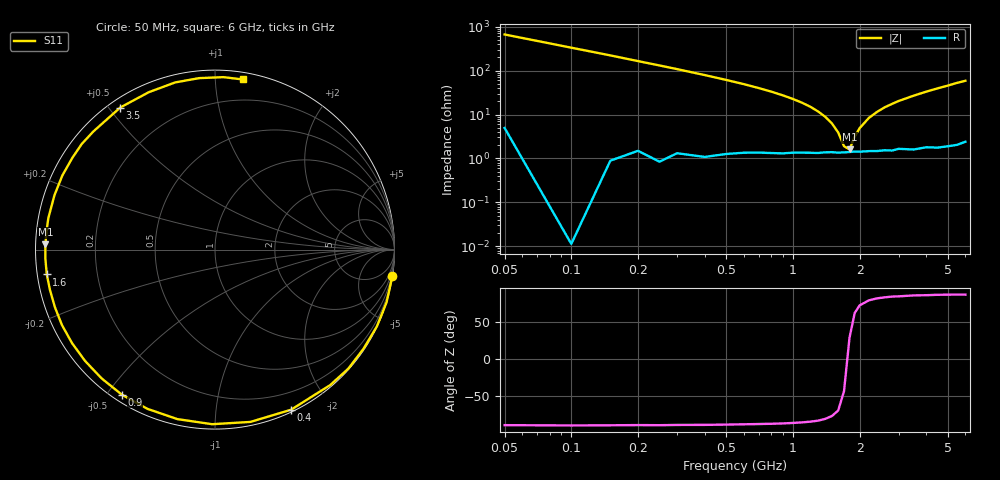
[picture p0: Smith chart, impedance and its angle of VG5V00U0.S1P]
! Infineon Technologies  Discrete & RF Semiconductors
! BB 831
! Si Tuning Diode in SOD323
! VR = 5 V
! S-Parameters:  July  1999
# GHz  S  MA  R  50
!  f  S11
! GHz  MAG  ANG
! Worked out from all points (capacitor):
!   34 points, 50 MHz to 6 GHz, reference 50 ohm
!   read as one part to ground: C = 4.77 pF near 50 MHz
!   lowest |Z| = 1.6 ohm at 1.8 GHz (marker M1)
!   series resonance near 1.763 GHz, so ESL is about 1.7 nH
!   S11 on the Smith chart (normalised r, x): 50 MHz: 0, -13; 400 MHz: 0.02, -1.58; 900 MHz: 0.03, -0.55; 1.6 GHz: 0.03, -0.07; 3.5 GHz: 0.03, +0.53; 6 GHz: 0.05, +1.17
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0.05  0.9989 -8.6
0.1  1 -17.1
0.15  0.9983 -25.4
0.25  0.9957 -41.8
0.3  0.9908 -49.6
0.4  0.9877 -64.6
0.5  0.98 -78.4
0.6  0.9729 -90.9
0.7  0.9675 -102.5
0.8  0.9637 -113.0
0.9  0.9606 -122.7
1  0.956 -131.4
1.1  0.9534 -139.4
1.2  0.9518 -146.8
1.4  0.9479 -160.2
1.6  0.9475 -171.6
1.8  0.9456 178.2
2  0.945 169.3
2.2  0.9444 161.3
2.4  0.9454 154.2
2.6  0.945 147.4
3  0.9447 135.8
3.5  0.9516 123.7
4  0.9514 112.8
4.5  0.9575 103.4
5  0.9594 95.3
5.5  0.962 87.2
6  0.9605 80.8
